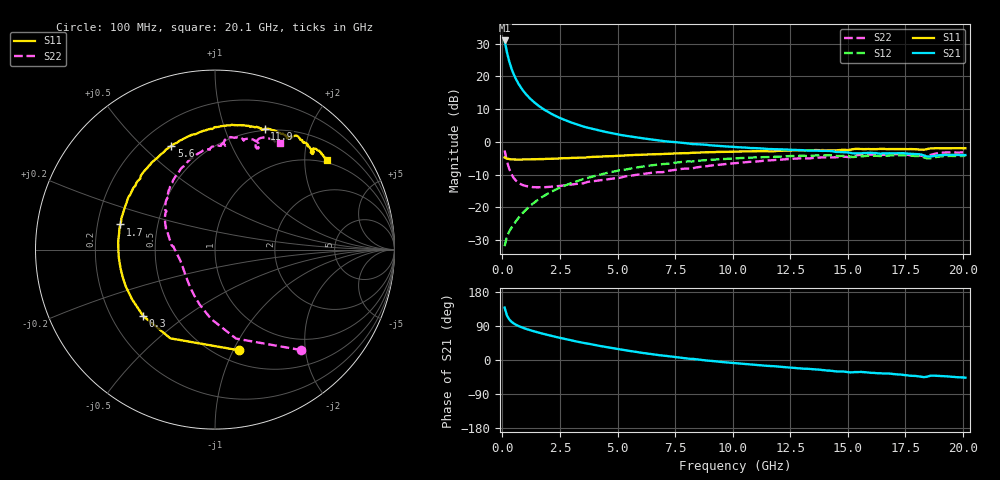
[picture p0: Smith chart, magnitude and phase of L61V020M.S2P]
!  Infineon Technologies AG
! BFR380L3 , PF131585-7, No.6, Th 09.10.01, soldered on pcb-board, measured with PP GSG850
!  Vce=1.0 V,  Ic=20.0 mA
! Common Emitter S-Parameters:  15. November 2001
#  GHz  S  MA  R  50
! f  S11  S21  S12  S22
! GHz  Mag  Ang  Mag  Ang  Mag  Ang  Mag  Ang
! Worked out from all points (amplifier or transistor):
!   201 points, 100 MHz to 20.1 GHz, reference 50 ohm
!   highest |S21| = 31.0 dB at 100 MHz (marker M1)
!   |S21| within 3 dB of that: start of sweep to 184.3 MHz
!   unconditionally stable (mu >= 1): 1.306 GHz to 4.867 GHz
!   at 3.4 GHz: K = 1.02, MAG = 7.4 dB, |S12| = -11.6 dB
!   at 10.1 GHz: K = 0.97, MSG = 1.7 dB, |S12| = -5.0 dB
!   at 20.1 GHz: K = 0.99, MSG = 0.1 dB, |S12| = -4.3 dB
!   S11 on the Smith chart (normalised r, x): 100 MHz: 0.63, -1.06; 300 MHz: 0.34, -0.35; 1.7 GHz: 0.30, +0.12; 5.6 GHz: 0.32, +0.62; 11.9 GHz: 0.48, +1.38; 20.1 GHz: 0.92, +2.56
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0.1  0.5777 -76.4  35.52 138.3  0.02545 61.3  0.7388 -49.3
0.2  0.5534 -116.7  23.58 117.6  0.03566 52.4  0.5094 -76.7
0.3  0.545 -137.2  17 107.3  0.0426 51.8  0.3865 -93.3
0.4  0.5388 -149.3  13.16 100.9  0.04888 53.7  0.3192 -105.3
0.5  0.5379 -157.6  10.7 96.3  0.05512 55.8  0.2793 -114.7
0.6  0.5366 -163.8  8.998 92.9  0.06185 57.6  0.2543 -122.2
0.7  0.5367 -168.7  7.771 89.8  0.06866 59.0  0.2377 -128.6
0.8  0.5363 -172.7  6.831 87.2  0.07564 60.3  0.2259 -133.9
1  0.5378 -179.0  5.511 82.8  0.08984 61.9  0.2124 -142.5
1.2  0.541 175.7  4.623 78.8  0.1044 62.6  0.2059 -149.1
1.4  0.5414 171.2  3.987 75.3  0.1192 62.8  0.2028 -154.5
1.7  0.5457 165.1  3.315 70.3  0.1415 62.3  0.2026 -160.9
2.1  0.5518 158.0  2.72 64.2  0.1707 60.9  0.2064 -167.5
2.5  0.5584 151.7  2.32 58.5  0.1996 58.9  0.212 -173.2
3.5  0.5743 137.1  1.727 45.4  0.2693 52.6  0.2318 175.7
5.6  0.6272 112.8  1.208 23.3  0.3927 38.0  0.3054 154.5
6.8  0.6529 101.2  1.053 12.8  0.4523 29.3  0.3445 142.5
10.1  0.711 77.0  0.8355 -8.4  0.5595 8.1  0.4727 116.4
11.9  0.7271 67.6  0.7723 -16.9  0.5955 -2.3  0.5301 102.8
13.5  0.7465 60.0  0.737 -24.4  0.6156 -11.7  0.5677 92.4
16.8  0.7769 47.8  0.6695 -35.9  0.6175 -26.8  0.6438 73.5
20.1  0.7999 38.6  0.6292 -46.6  0.6116 -39.9  0.6929 58.6
